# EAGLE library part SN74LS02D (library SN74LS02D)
HEX INVERTERS Source: Datasheet
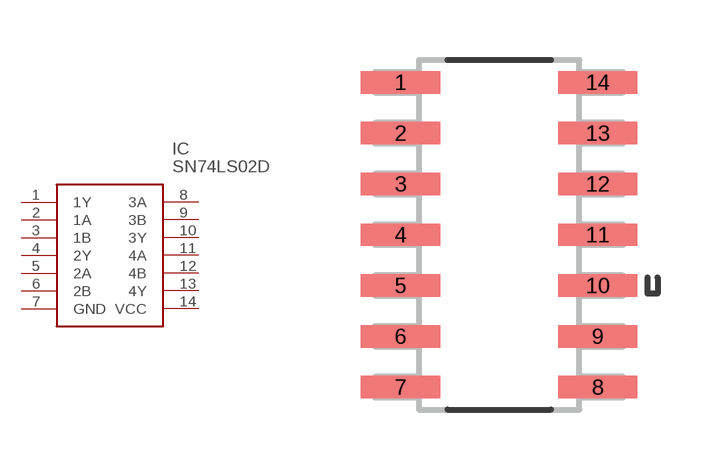
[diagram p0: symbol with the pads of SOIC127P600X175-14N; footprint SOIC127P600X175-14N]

Designator prefix IC

## SN74LS02D (Description: HEX INVERTERS; Height: mm; Manufacturer_Name: Texas Instruments; Manufacturer_Part_Number: SN74LS02D; Mouser_Part_Number: 595-SN74LS02D; Mouser_Price-Stock: https://www.mouser.com/Search/Refine.aspx?Keyword=595-SN74LS02D; RS_Part_Number: 6632357P; RS_Price-Stock: http://uk.rs-online.com/web/p/products/6632357P)  [SOIC127P600X175-14N]
1  1Y
2  1A
3  1B
4  2Y
5  2A
6  2B
7  GND
8  3A
9  3B
10  3Y
11  4A
12  4B
13  4Y
14  VCC

## Footprint SOIC127P600X175-14N (pad centres in mm)
SOIC127P600X175-14N
smd 1.981 x 0.559: 1 -2.464,3.81; 2 -2.464,2.54; 3 -2.464,1.27; 4 -2.464,0; 5 -2.464,-1.27; 6 -2.464,-2.54; 7 -2.464,-3.81; 8 2.464,-3.81; 9 2.464,-2.54; 10 2.464,-1.27; 11 2.464,0; 12 2.464,1.27; 13 2.464,2.54; 14 2.464,3.81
